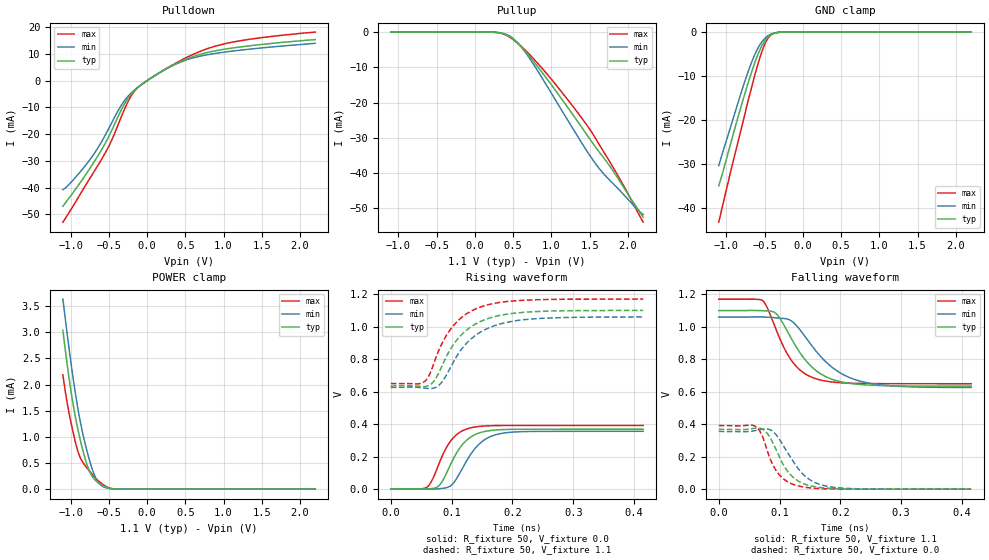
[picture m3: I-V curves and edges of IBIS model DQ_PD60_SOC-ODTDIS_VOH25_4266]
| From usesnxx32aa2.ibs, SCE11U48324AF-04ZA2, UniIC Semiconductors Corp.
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| DQ_PD60_SOC-ODTDIS_VOH25_4266
| (60 Ohm Pulldown, SOC ODT disabled setting, VOH=VDDQ/2.5 cal. point, 3200-4266Mbps)
[Model]   DQ_PD60_SOC-ODTDIS_VOH25_4266
Model_type   I/O
Vinl = 160.000mV
Vinh = 280.000mV
Vmeas = 220.000mV
Vref = 0.0mV
Cref = 0.0pF
|   typ   min   max
|C_comp   0.797pF   0.747pF   0.847pF
C_comp_pullup   0.3985pF   0.3735pF   0.4235pF
C_comp_pulldown   0.3985pF   0.3735pF   0.4235pF
| Note: C_comp changes when the ODT circuit is enabled.
[Model Spec]
| Input threshold voltage corners
Vinl   0.1600V   0.1520V   0.1740V
Vinh   0.2800V   0.2720V   0.2940V
| Measurement voltage corners
Vmeas   0.2200V   0.2120V   0.2340V
| Timing spec test load voltage corners
Vref   0.0000V   0.0000V   0.0000V
| Dynamic Overshoot Parameters from LPDDR4 Specification
D_overshoot_ampl_h   0.30   NA   NA
D_overshoot_ampl_l   0.30   NA   NA
D_overshoot_area_h   0.1n   NA   NA
D_overshoot_area_l   0.1n   NA   NA
[Receiver Thresholds]
Vth   = 0.2200V
Vth_min  = 0.2167V
Vth_max  = 0.2233V
Vinh_ac  = 0.060V
Vinh_dc  = 0.060V
Vinl_ac  = -0.060V
Vinl_dc  = -0.060V
Tslew_ac = 5.000ns |Not specified, so set to high value
Threshold_sensitivity = 0.2000
Reference_supply Pullup_ref
[Voltage Range]   1.1000V   1.0600V   1.1700V
[Pullup Reference]   1.1000V   1.0600V   1.1700V
| Junction Temperature (Ambient temp is 35C typ 95C min -40C max)
[Temperature Range]   50.0   110.0   -40.0
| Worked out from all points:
|   slope of the pulldown table from 0 to 0.165 V, typ, clamps not added: 54.7 ohm
|   slope of the pullup table from 0 to 0.165 V, typ, clamps not added: 17.2 kohm
|   GND clamp passes 1 mA (typ) near -0.45 V on its own axis
|   POWER clamp passes 1 mA (typ) near -0.88 V on its own axis
|   rising waveform, R_fixture 50, V_fixture 0.0: 20-80 % time 34.5ps typ, 38.2ps min, 31.3ps max; typ from 0.001 V to 0.369 V
|   falling waveform, R_fixture 50, V_fixture 1.1: 20-80 % time 53.1ps typ, 65.9ps min, 42.5ps max; typ from 1.1 V to 0.635 V
|   rising waveform, R_fixture 50, V_fixture 1.1: 20-80 % time 54.5ps typ, 57.4ps min, 50.7ps max; typ from 0.635 V to 1.1 V
|   falling waveform, R_fixture 50, V_fixture 0.0: 20-80 % time 34.4ps typ, 41.3ps min, 29ps max; typ from 0.369 V to 0.001 V
[Pulldown]
|   Voltage   I(typ)   I(min)   I(max)
-1.1V     -46.99mA   -40.8mA    -52.96mA
-786.5mV  -34.49mA   -31.05mA   -38.36mA
-641.3mV  -28.08mA   -25.11mA   -31.66mA
-525.8mV  -22.32mA   -19.3mA    -25.97mA
-360.8mV  -12.37mA   -10.39mA   -15.26mA
-261.8mV  -7.137mA   -6.288mA   -8.642mA
-176mV    -4.016mA   -3.794mA   -4.406mA
-80.3mV   -1.664mA   -1.635mA   -1.657mA
411.4mV   6.783mA    6.597mA    7.102mA
847mV     10.89mA    9.975mA    12.5mA
1.375V    13.14mA    11.88mA    15.61mA
2.2V      15.36mA    13.96mA    18.16mA
[GND Clamp]
|   Voltage   I(typ)   I(min)   I(max)
-1.1V     -34.89mA   -30.34mA   -43.14mA
-941.6mV  -25.14mA   -21.33mA   -31.48mA
-786.5mV  -15.6mA    -12.65mA   -20.6mA
-720.5mV  -11.8mA    -9.214mA   -15.96mA
-661.1mV  -8.6mA     -6.453mA   -11.91mA
-585.2mV  -4.992mA   -3.582mA   -7.141mA
-519.2mV  -2.574mA   -1.836mA   -3.675mA
-466.4mV  -1.312mA   -948.2uA   -1.694mA
-413.6mV  -570.8uA   -419.7uA   -620.3uA
-350.9mV  -170.2uA   -127.7uA   -146.8uA
-258.5mV  -16.58uA   -14.44uA   -9.815uA
2.2V      0A         0A         0A
[Pullup]
|   Voltage   I(typ)   I(min)   I(max)
-1.1V     4.112uA    7.441uA    1.363uA
262.9mV   -64.84uA   -63.6uA    -66.39uA
398.2mV   -661.4uA   -551.1uA   -783.7uA
510.4mV   -2.22mA    -2.012mA   -2.306mA
612.7mV   -4.381mA   -4.395mA   -4.2mA
751.3mV   -7.908mA   -8.649mA   -7.214mA
1.055V    -16.59mA   -19.32mA   -14.85mA
1.441V    -28.41mA   -32.96mA   -25.69mA
1.576V    -32.59mA   -37.31mA   -30.11mA
1.698V    -36.11mA   -40.55mA   -34.5mA
1.956V    -44.42mA   -46.36mA   -44.02mA
2.2V      -52.46mA   -51.75mA   -53.91mA
[POWER Clamp]
|   Voltage   I(typ)   I(min)   I(max)
-1.1V     3.036mA    3.636mA    2.186mA
-1.041V   2.347mA    2.931mA    1.626mA
-977.9mV  1.724mA    2.242mA    1.161mA
-908.6mV  1.178mA    1.582mA    748.3uA
-852.5mV  818.5uA    1.149mA    543.8uA
-776.6mV  434.4uA    683.6uA    390.2uA
-713.9mV  239.2uA    373.1uA    278.6uA
-654.5mV  142.7uA    170.4uA    185.9uA
-598.4mV  83.67uA    71.97uA    113uA
-502.7mV  22.64uA    14.15uA    29.28uA
-390.5mV  2.096uA    1.409uA    1.763uA
2.2V      0A         0A         0A
[Ramp]
|   typ   min   max
| 20% - 80%
dV/dt_r   220.76m/34.45p   213.10m/38.18p   234.84m/31.31p
dV/dt_f   279.06m/53.10p   260.18m/65.93p   312.25m/42.55p
| 25% - 75%
|dV/dt_r   183.97m/27.42p   177.58m/30.41p   195.70m/24.82p
|dV/dt_f   232.55m/42.27p   216.82m/52.42p   260.21m/33.82p
R_load = 50
[Rising Waveform]
R_fixture = 50
V_fixture = 0.0
|   Time   V(typ)   V(min)   V(max)
0s        726.5uV    592.8uV    533uV
58ps      587.8uV    -78.52uV   8.289mV
67ps      3.282mV    -514.6uV   48.79mV
77ps      14.06mV    1.164mV    135mV
101ps     173.3mV    28.69mV    308.2mV
115ps     261.3mV    108.9mV    353.3mV
130ps     316.9mV    206.7mV    376.1mV
155ps     355.3mV    305.8mV    388.8mV
187ps     366.8mV    345.9mV    391.6mV
415ps     368.7mV    355.8mV    391.9mV
[Falling Waveform]
R_fixture   = 50
V_fixture   = 1.1
V_fixture_min = 1.06
V_fixture_max = 1.17
|   Time   V(typ)   V(min)   V(max)
0s        1.1V       1.06V      1.17V
73ps      1.099V     1.061V     1.159V
95ps      1.079V     1.055V     976.9mV
118ps     937.6mV    1.04V      801.6mV
136ps     827.5mV    970.3mV    726.7mV
157ps     739.9mV    864.5mV    683.6mV
191ps     671.3mV    737.7mV    658.6mV
233ps     644.6mV    664.8mV    651.4mV
291ps     636.5mV    634.5mV    649.8mV
415ps     634.9mV    626.4mV    649.6mV
[Rising Waveform]
R_fixture   = 50
V_fixture   = 1.1
V_fixture_min = 1.06
V_fixture_max = 1.17
|   Time   V(typ)   V(min)   V(max)
0s        634.8mV    625.9mV    649.6mV
54ps      630.8mV    622.1mV    658.5mV
63ps      638.8mV    618.9mV    700mV
76ps      694.2mV    630.8mV    827.5mV
90ps      805.9mV    692.7mV    937.6mV
108ps     915.3mV    815.8mV    1.028V
126ps     983.1mV    903.7mV    1.083V
148ps     1.033V     967.9mV    1.122V
227ps     1.091V     1.046V     1.164V
415ps     1.1V       1.06V      1.17V
[Falling Waveform]
R_fixture = 50
V_fixture = 0.0
|   Time   V(typ)   V(min)   V(max)
0s        368.8mV    355.9mV    392mV
57ps      374.7mV    359.2mV    392.6mV
73ps      368.3mV    370.8mV    315.2mV
85ps      313.9mV    365.4mV    183.1mV
96ps      230.2mV    327.7mV    106.3mV
112ps     116.8mV    233.1mV    49.02mV
130ps     52.26mV    130.3mV    20.92mV
155ps     17.58mV    47.19mV    6.762mV
190ps     4.405mV    11.53mV    1.759mV
415ps     771.1uV    658.5uV    552uV
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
